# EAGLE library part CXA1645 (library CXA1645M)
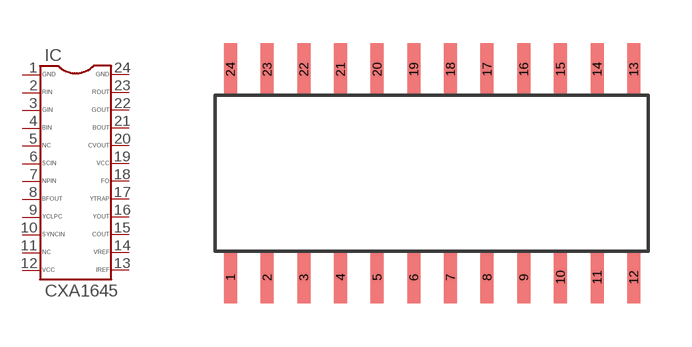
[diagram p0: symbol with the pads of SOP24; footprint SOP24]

Designator prefix IC

## CXA1645  [SOP24]
1  1  pas
2  2  pas
3  3  pas
4  4  pas
5  5  pas
6  6  pas
7  7  pas
8  8  pas
9  9  pas
10  10  pas
11  11  pas
12  12  pas
13  13  pas
14  14  pas
15  15  pas
16  16  pas
17  17  pas
18  18  pas
19  19  pas
20  20  pas
21  21  pas
22  22  pas
23  23  pas
24  24  pas

## Footprint SOP24 (pad centres in mm)
smd 0.45 x 1.8: 1 -6.97,-3.6; 2 -5.7,-3.6; 3 -4.43,-3.6; 4 -3.16,-3.6; 5 -1.89,-3.6; 6 -0.62,-3.6; 7 0.65,-3.6; 8 1.92,-3.6; 9 3.19,-3.6; 10 4.46,-3.6; 11 5.73,-3.6; 12 7,-3.6; 13 7,3.6; 14 5.73,3.6; 15 4.46,3.6; 16 3.19,3.6; 17 1.92,3.6; 18 0.65,3.6; 19 -0.62,3.6; 20 -1.89,3.6; 21 -3.16,3.6; 22 -4.43,3.6; 23 -5.7,3.6; 24 -6.97,3.6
